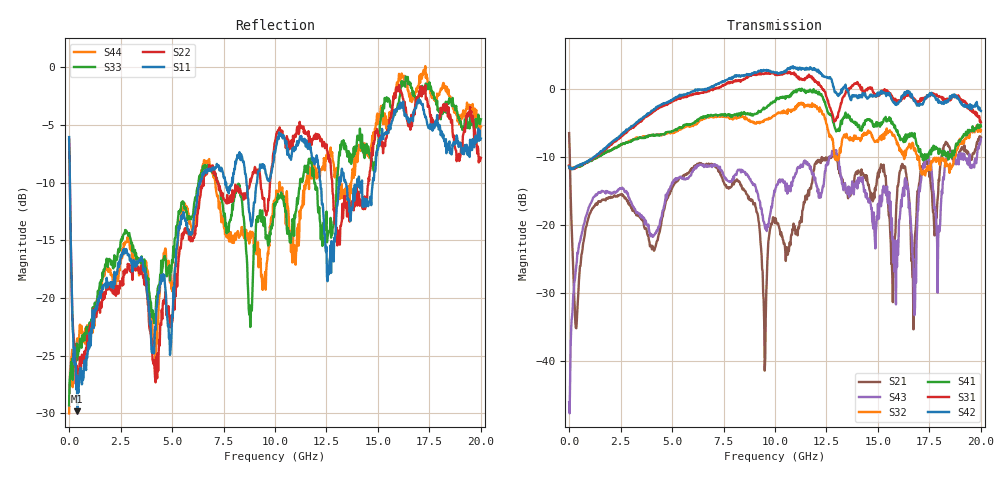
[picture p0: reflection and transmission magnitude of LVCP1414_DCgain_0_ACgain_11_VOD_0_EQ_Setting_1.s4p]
!Agilent Technologies,N5230A,MY46400459,A.07.50.48
!Agilent N5230A: A.07.50.48
!Date: Tuesday, April 17, 2012 18:37:00
!Correction: S11(Full 4 Port(1,2,3,4))
!S12(Full 4 Port(1,2,3,4))
!S13(Full 4 Port(1,2,3,4))
!S14(Full 4 Port(1,2,3,4))
!S21(Full 4 Port(1,2,3,4))
!S22(Full 4 Port(1,2,3,4))
!S23(Full 4 Port(1,2,3,4))
!S24(Full 4 Port(1,2,3,4))
!S31(Full 4 Port(1,2,3,4))
!S32(Full 4 Port(1,2,3,4))
!S33(Full 4 Port(1,2,3,4))
!S34(Full 4 Port(1,2,3,4))
!S41(Full 4 Port(1,2,3,4))
!S42(Full 4 Port(1,2,3,4))
!S43(Full 4 Port(1,2,3,4))
!S44(Full 4 Port(1,2,3,4))
!S4P File: Measurements: <S11,S12,S13,S14>,
!<S21,S22,S23,S24>,
!<S31,S32,S33,S34>,
!<S41,S42,S43,S44>:
# Hz S  dB  R 50
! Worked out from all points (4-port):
!   801 points, 300 kHz to 20 GHz, reference 50 ohm
!   strongest paths, dB at 300 kHz, 5 GHz, 10 GHz, 15 GHz, 20 GHz:
!     S42: -11.4, -1.5, 2.4, -0.5, -3.2
!     S31: -11.2, -1.8, 2.1, -1.0, -4.9
!     S41: -11.3, -6.2, -1.9, -5.4, -5.5
!     S32: -11.4, -6.4, -3.9, -7.8, -6.1
!     S43: -46.1, -13.8, -15.1, -16.9, -7.3
!     S21: -6.5, -14.6, -19.7, -12.3, -7.1
!   lowest |S11| = -29.8 dB at 400.3 MHz (marker M1), VSWR 1.07, Z = 52.9 + j1.59 ohm
!   |S11| at or under -10 dB: 37.51 MHz to 6.362 GHz (6.324 GHz wide, 198 % of centre); 12.21 GHz to 13.11 GHz (907 MHz wide, 7.17 % of centre); 13.44 GHz to 13.99 GHz (542.8 MHz wide, 3.96 % of centre)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
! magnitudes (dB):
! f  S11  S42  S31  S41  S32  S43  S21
! 300 kHz  -6.0  -11.4  -11.2  -11.3  -11.4  -46.1  -6.5
! 400.3 MHz  -29.8  -11.3  -11.4  -11.4  -11.4  -24.1  -32.4
! 10.03 GHz  -7.2  2.4  2.2  -1.6  -3.8  -14.6  -19.0
! 12.73 GHz  -17.8  1.5  -3.2  -3.9  -6.9  -9.9  -9.9
! 16.8 GHz  -3.5  -1.7  -1.5  -7.1  -8.7  -32.2  -21.6
! 17.38 GHz  -4.7  -1.1  -0.9  -9.6  -12.1  -10.4  -10.7
! 20 GHz  -6.2  -3.2  -4.9  -5.5  -6.1  -7.3  -7.1
